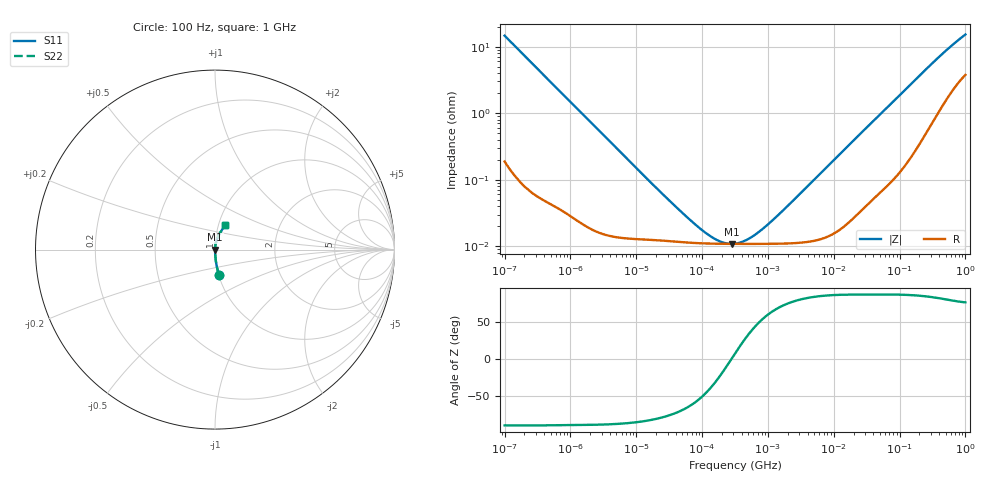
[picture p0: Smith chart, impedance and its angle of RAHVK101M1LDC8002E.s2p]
! RAHVK101M1LDC8002E  S-PARAMETER MODEL  (AEC-Q200 qualified)
! Model Generated by ELNA Corporation (http://www.ty-top.com)
! Version 1.0
! ELNA Control No. 201029
! Copyright (c) 2020 ELNA CO.,LTD. All Rights Reserved.
! Products Name : CONDUCTIVE POLYMER HYBRID ALUMINUM ELECTROLYTIC CAPACITORS
! Characteristics :
!  Capacitance  :  100uF  ,  Rated voltage  :  10V
!  Operating Temp. Range  :  -55 to +125 degC  ,  Endurance  :  4000hr at 125 degC
!  Dimension D  :  6.3mm  ,  Dimension L  :  5.8mm
! Frequency Range : 100Hz - 1GHz
! External Node Assignments :
!  1  o---| |---o  2
# MHz S RI R 50
!Freq[MHz].  S11 Real  S11 Imag  S21 Real  S21 Imag  S12 Real  S12 Imag  S22 Real  S22 Imag
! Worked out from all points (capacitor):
!   401 points, 100 Hz to 1 GHz, reference 50 ohm
!   read as one part in series: C = 109 uF near 108 Hz
!   lowest |Z| = 10.9 mohm at 280.2 kHz (marker M1)
!   series resonance near 280.3 kHz, so ESL is about 3 nH
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0.0001  0.0227 -0.1425  0.9773 0.1425  0.9773 0.1425  0.0227 -0.1425
0.000113  0.018 -0.1269  0.982 0.1269  0.982 0.1269  0.018 -0.1269
0.000183  0.00719 -0.0792  0.9928 0.0792  0.9928 0.0792  0.00719 -0.0792
0.000309  0.0028 -0.0472  0.9972 0.0472  0.9972 0.0472  0.0028 -0.0472
0.001488  0.000318 -0.00996  0.9997 0.00996  0.9997 0.00996  0.000318 -0.00996
0.022131  0.000123 -0.000676  0.9999 0.000676  0.9999 0.000676  0.000123 -0.000676
0.060604  0.000114 -0.000242  0.9999 0.000242  0.9999 0.000242  0.000114 -0.000242
0.115478  0.00011 -0.000112  0.9999 0.000112  0.9999 0.000112  0.00011 -0.000112
0.187284  0.000109 -4.6e-05  0.9999 4.6e-05  0.9999 4.6e-05  0.000109 -4.6e-05
0.229087  0.000109 -2.26e-05  0.9999 2.26e-05  0.9999 2.26e-05  0.000109 -2.26e-05
0.280221  0.000109 -3.3e-08  0.9999 3.3e-08  0.9999 3.3e-08  0.000109 -3.3e-08
0.316228  0.000109 1.34e-05  0.9999 -1.34e-05  0.9999 -1.34e-05  0.000109 1.34e-05
0.386812  0.000108 3.64e-05  0.9999 -3.64e-05  0.9999 -3.64e-05  0.000108 3.64e-05
0.492606  0.000108 6.61e-05  0.9999 -6.61e-05  0.9999 -6.61e-05  0.000108 6.61e-05
0.798914  0.000109 0.000139  0.9999 -0.000139  0.9999 -0.000139  0.000109 0.000139
1.522299  0.000109 0.000292  0.9999 -0.000292  0.9999 -0.000292  0.000109 0.000292
4.704354  0.00012 0.000929  0.9999 -0.000929  0.9999 -0.000929  0.00012 0.000929
69.9842  0.00104 0.013  0.999 -0.013  0.999 -0.013  0.00104 0.013
176.8072  0.00382 0.032  0.9962 -0.032  0.9962 -0.032  0.00382 0.032
395.8221  0.015 0.0672  0.985 -0.0672  0.985 -0.0672  0.015 0.0672
695.825  0.0354 0.105  0.9646 -0.105  0.9646 -0.105  0.0354 0.105
1000  0.0553 0.1343  0.9447 -0.1343  0.9447 -0.1343  0.0553 0.1343
